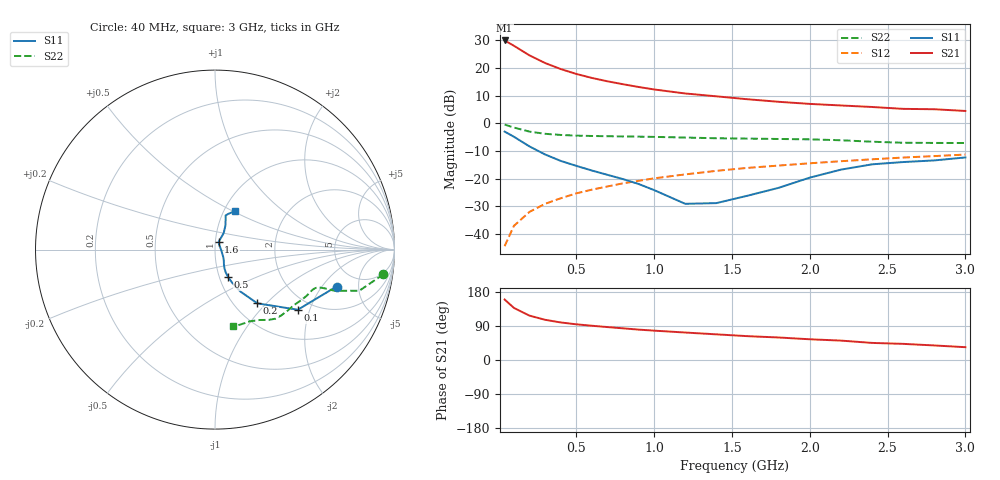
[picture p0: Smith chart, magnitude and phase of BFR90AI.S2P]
! Filename:  BFR90AI.S2P  Version:  2.0
! Philips part #: BFR90A  Date: Jul 1990
! Bias condition: Vce=10V, Ic=15mA
#  MHz  S  MA  R  50
! Freq  S11  S21  S12  S22  !GUM [dB]
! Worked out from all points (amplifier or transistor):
!   21 points, 40 MHz to 3 GHz, reference 50 ohm
!   highest |S21| = 29.9 dB at 40 MHz (marker M1)
!   |S21| within 3 dB of that: start of sweep to 130.8 MHz
!   unconditionally stable (mu >= 1): 591.2 MHz to end of sweep
!   at 300 MHz: K = 0.88, MSG = 25.5 dB, |S12| = -29.1 dB
!   at 1 GHz: K = 1.05, MAG = 14.7 dB, |S12| = -19.9 dB
!   at 3 GHz: K = 1.09, MAG = 6.0 dB, |S12| = -11.3 dB
!   S11 on the Smith chart (normalised r, x): 40 MHz: 3.41, -2.81; 100 MHz: 1.68, -1.66; 200 MHz: 1.27, -0.89; 500 MHz: 1.10, -0.35; 1.6 GHz: 1.04, +0.09; 3 GHz: 1.12, +0.51
40  0.708 -16.9  31.41 159.6  0.006 81.6  0.948 -8.4
100  0.57 -36.0  25.16 137.4  0.014 75.1  0.836 -15.9
200  0.381 -51.8  16.85 117.0  0.025 73.3  0.706 -19.0
300  0.273 -58.8  12.28 106.1  0.035 73.8  0.645 -19.5
400  0.209 -62.5  9.559 99.1  0.044 75.2  0.615 -20.0
500  0.17 -64.6  7.798 94.2  0.054 75.6  0.598 -21.0
600  0.14 -64.8  6.603 90.4  0.063 75.2  0.589 -22.2
700  0.117 -63.2  5.742 86.9  0.072 75.2  0.583 -23.5
800  0.098 -59.4  5.081 83.6  0.082 74.8  0.578 -25.0
900  0.08 -52.1  4.531 80.2  0.091 74.4  0.573 -26.4
1000  0.062 -42.1  4.085 77.5  0.101 73.7  0.567 -27.9
1200  0.035 -5.5  3.457 72.5  0.119 72.4  0.552 -31.5
1400  0.036 50.4  3.07 67.7  0.138 71.0  0.536 -35.7
1600  0.049 65.0  2.718 62.9  0.156 69.6  0.528 -40.5
1800  0.068 63.4  2.445 59.4  0.172 68.3  0.52 -45.0
2000  0.104 62.2  2.239 54.7  0.189 66.7  0.512 -48.7
2200  0.145 66.5  2.098 51.2  0.206 65.1  0.493 -52.6
2400  0.181 70.8  1.97 45.1  0.223 63.4  0.464 -57.7
2600  0.199 72.8  1.821 42.6  0.24 61.3  0.444 -64.2
2800  0.213 69.4  1.793 38.4  0.255 59.9  0.441 -71.2
3000  0.241 62.8  1.67 33.8  0.272 59.1  0.44 -76.7
